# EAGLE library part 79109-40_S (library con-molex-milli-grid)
RECEPTACAL
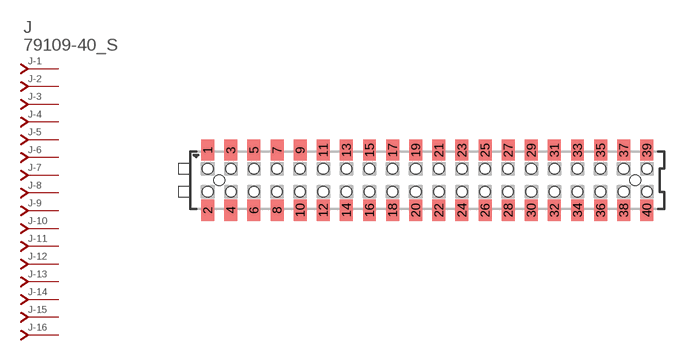
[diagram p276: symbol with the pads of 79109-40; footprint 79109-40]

Designator prefix J; gates -1=J-NV -2=J-N -3=J-N -4=J-N -5=J-N -6=J-N -7=J-N -8=J-N -9=J-N -10=J-N -11=J-N -12=J-N -13=J-N -14=J-N -15=J-N -16=J-N -17=J-N -18=J-N -19=J-N -20=J-N -21=J-N -22=J-N -23=J-N -24=J-N -25=J-N -26=J-N -27=J-N -28=J-N -29=J-N -30=J-N -31=J-N -32=J-N -33=J-N -34=J-N -35=J-N -36=J-N -37=J-N -38=J-N -39=J-N -40=J-N

## 79109-40_S  [79109-40]
1  -1:J  pas
2  -2:J  pas
3  -3:J  pas
4  -4:J  pas
5  -5:J  pas
6  -6:J  pas
7  -7:J  pas
8  -8:J  pas
9  -9:J  pas
10  -10:J  pas
11  -11:J  pas
12  -12:J  pas
13  -13:J  pas
14  -14:J  pas
15  -15:J  pas
16  -16:J  pas
17  -17:J  pas
18  -18:J  pas
19  -19:J  pas
20  -20:J  pas
21  -21:J  pas
22  -22:J  pas
23  -23:J  pas
24  -24:J  pas
25  -25:J  pas
26  -26:J  pas
27  -27:J  pas
28  -28:J  pas
29  -29:J  pas
30  -30:J  pas
31  -31:J  pas
32  -32:J  pas
33  -33:J  pas
34  -34:J  pas
35  -35:J  pas
36  -36:J  pas
37  -37:J  pas
38  -38:J  pas
39  -39:J  pas
40  -40:J  pas

## Footprint 79109-40 (pad centres in mm)
RECEPTACAL SMD Dual Row, Vertical, Pass-Thru
smd 1.12 x 1.83: 1 -19,2.6; 2 -19,-2.6; 3 -17,2.6; 4 -17,-2.6; 5 -15,2.6; 6 -15,-2.6; 7 -13,2.6; 8 -13,-2.6; 9 -11,2.6; 10 -11,-2.6; 11 -9,2.6; 12 -9,-2.6; 13 -7,2.6; 14 -7,-2.6; 15 -5,2.6; 16 -5,-2.6; 17 -3,2.6; 18 -3,-2.6; 19 -1,2.6; 20 -1,-2.6; 21 1,2.6; 22 1,-2.6; 23 3,2.6; 24 3,-2.6; 25 5,2.6; 26 5,-2.6; 27 7,2.6; 28 7,-2.6; 29 9,2.6; 30 9,-2.6; 31 11,2.6; 32 11,-2.6; 33 13,2.6; 34 13,-2.6; 35 15,2.6; 36 15,-2.6; 37 17,2.6; 38 17,-2.6; 39 19,2.6; 40 19,-2.6
hole 0.914 at -18,0
hole 0.914 at -19,1
hole 0.914 at -19,-1
hole 0.914 at -17,-1
hole 0.914 at -17,1
hole 0.914 at -15,-1
hole 0.914 at -15,1
hole 0.914 at 18,0
hole 0.914 at -13,1
hole 0.914 at -13,-1
hole 0.914 at -11,1
hole 0.914 at -11,-1
hole 0.914 at -9,1
hole 0.914 at -9,-1
hole 0.914 at -7,1
hole 0.914 at -7,-1
hole 0.914 at -5,-1
hole 0.914 at -5,1
hole 0.914 at -3,1
hole 0.914 at -3,-1
hole 0.914 at -1,1
hole 0.914 at -1,-1
hole 0.914 at 1,1
hole 0.914 at 1,-1
hole 0.914 at 3,-1
hole 0.914 at 3,1
hole 0.914 at 5,1
hole 0.914 at 7,1
hole 0.914 at 9,1
hole 0.914 at 5,-1
hole 0.914 at 7,-1
hole 0.914 at 9,-1
hole 0.914 at 11,-1
hole 0.914 at 13,-1
hole 0.914 at 15,-1
hole 0.914 at 17,-1
hole 0.914 at 19,-1
hole 0.914 at 11,1
hole 0.914 at 13,1
hole 0.914 at 15,1
hole 0.914 at 17,1
hole 0.914 at 19,1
